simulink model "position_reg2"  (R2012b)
settings: Solver=ode45  StartTime=0.0  StopTime=10.0  RelTol=1e-3
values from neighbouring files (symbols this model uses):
  D = 10    [position_reg_1.m]    (also in position_reg_2.m; rad_aufhaeng_3.m = [0;ct]; rad_aufhaeng_4.m = [0;ct])
  FG = 500    [coulomb_1.m]    (also in coulomb_10.m = 10; coulomb_11.m = 10; coulomb_2.m; coulomb_3.m)
  FH = 12    [coulomb_10.m]    (also in coulomb_11.m; coulomb_3.m = 600; coulomb_4.m = 600; position_reg_1.m = 3.956)
  I = 20    [position_reg_1.m]    (also in position_reg_2.m; suspension_1.m = 225; suspension_2.m = 225; suspension_3.m = 225)
  m1 = 100    [feder_masse_1.m]    (also in feder_masse_11.m; feder_masse_13.m; feder_masse_14.m; position_reg_2.m = 1)
  P = 10    [position_reg_1.m]    (also in position_reg_2.m; vibration_control_1.m = em_ampl*i_ampl/2,; vibration_control_2.m = emf_ampl*i_ampl/2,; vibration_control_3.m = emf_ampl*i_ampl/2,)
  sigma_0 = 5000    [position_reg_1.m]    (also in position_reg_2.m; slip_stick_21.m = 10000; slip_stick_s_12.m = 10000; tilger_gleitreib2.m = 1000)
  sigma_1 = sqrt(sigma_0)    [position_reg_1.m]    (also in position_reg_2.m; slip_stick_21.m = sqrt(1e5); slip_stick_s_12.m = sqrt(1e5); tilger_gleitreib2.m)
  sigma_2 = 0    [position_reg_1.m]    (also in position_reg_2.m; slip_stick_21.m; slip_stick_s_12.m; tilger_gleitreib2.m)
  vs = 0.05    [position_reg_1.m]    (also in position_reg_2.m; slip_stick_21.m; slip_stick_3.m = 0.01; slip_stick_31.m)
libraries: simulink x1

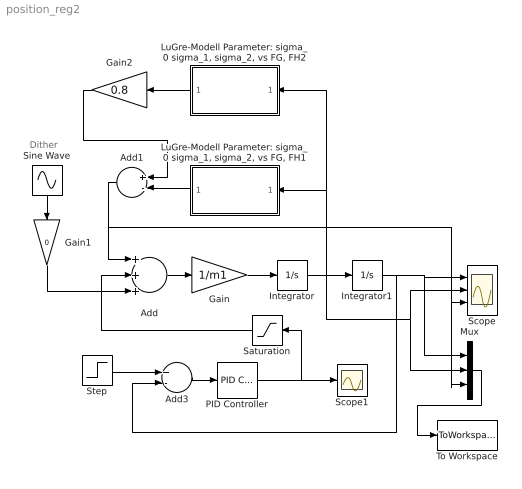
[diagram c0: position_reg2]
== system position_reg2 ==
  note: Dither
  Add : Sum  Inputs=+++
  Add1 : Sum  Inputs=+-
  Add3 : Sum  Inputs=+-
  Gain : Gain  Gain=1/m1
  Gain1 : Gain  Gain=0
  Gain2 : Gain  Gain=0.8
  Integrator : Integrator
  Integrator1 : Integrator
  "LuGre-Modell Parameter: sigma_0 sigma_1, sigma_2, vs FG, FH1" : Subsystem
  "LuGre-Modell Parameter: sigma_0 sigma_1, sigma_2, vs FG, FH2" : Subsystem
  Mux : Mux  Inputs=3
  PID Controller : simulink/Continuous/PID Controller  Controller=PID  TimeDomain=Continuous-time  SampleTime=1  IntegratorMethod=Forward Euler  FilterMethod=Forward Euler  Form=Parallel  P=P  I=I  D=D  N=100  InitialConditionSource=internal  InitialConditionForIntegrator=0  InitialConditionForFilter=0  ExternalReset=none  LimitOutput=off  UpperSaturationLimit=inf  LowerSaturationLimit=-inf  LinearizeAsGain=on  AntiWindupMode=none  Kb=1  TrackingMode=off  Kt=1  PParamMin=[]  PParamMax=[]  IParamMin=[]  IParamMax=[]  DParamMin=[]  DParamMax=[]  NParamMin=[]  NParamMax=[]  KbParamMin=[]  KbParamMax=[]  KtParamMin=[]  KtParamMax=[]  POutMin=[]  POutMax=[]  IOutMin=[]  IOutMax=[]  DOutMin=[]  DOutMax=[]  NOutMin=[]  NOutMax=[]  KbOutMin=[]  KbOutMax=[]  KtOutMin=[]  KtOutMax=[]  IntegratorOutMin=[]  IntegratorOutMax=[]  FilterOutMin=[]  FilterOutMax=[]  SumOutMin=[]  SumOutMax=[]  SumI1OutMin=[]  SumI1OutMax=[]  SumI2OutMin=[]  SumI2OutMax=[]  SumI3OutMin=[]  SumI3OutMax=[]  SumDOutMin=[]  SumDOutMax=[]  SaturationOutMin=[]  SaturationOutMax=[]  IntegratorContinuousStateAttributes=''  IntegratorStateMustResolveToSignalObject=off  IntegratorRTWStateStorageClass=Auto  FilterContinuousStateAttributes=''  FilterStateMustResolveToSignalObject=off  FilterRTWStateStorageClass=Auto
  Saturation : Saturate  UpperLimit=5  LowerLimit=-5  ZeroCross=off
  Scope : Scope  NumInputPorts=3
  Scope1 : Scope
  Sine Wave : Sin  Amplitude=4  Frequency=30  SampleTime=0
  Step : Step  Time=0  SampleTime=0
  To Workspace : ToWorkspace  VariableName=y  SampleTime=-1  SaveFormat=Structure With Time
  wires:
  Add/1 -> Gain/1
  Gain/1 -> Integrator/1
  Integrator/1 -> "LuGre-Modell Parameter: sigma_0 sigma_1, sigma_2, vs FG, FH1"/1(v), "LuGre-Modell Parameter: sigma_0 sigma_1, sigma_2, vs FG, FH2"/1(v), Mux/2, Scope/2, Integrator1/1
  Integrator1/1 -> Add3/2, Mux/1, Scope/1
  Add3/1 -> PID Controller/1
  Step/1 -> Add3/1
  "LuGre-Modell Parameter: sigma_0 sigma_1, sigma_2, vs FG, FH1"/1(Fr) -> Add1/2
  PID Controller/1 -> Saturation/1, Scope1/1
  Saturation/1 -> Add/2
  Sine Wave/1 -> Gain1/1
  Mux/1 -> To Workspace/1
  Gain1/1 -> Add/3
  "LuGre-Modell Parameter: sigma_0 sigma_1, sigma_2, vs FG, FH2"/1(Fr) -> Gain2/1
  Gain2/1 -> Add1/1
  Add1/1 -> Scope/3, Mux/3, Add/1

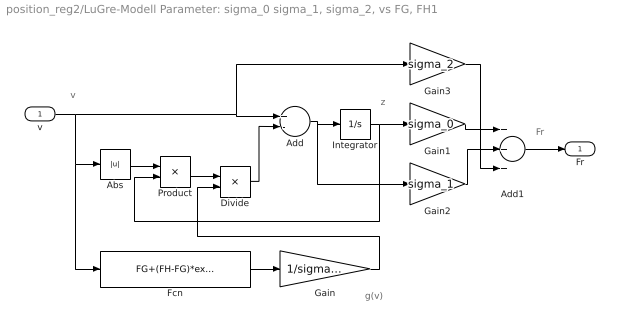
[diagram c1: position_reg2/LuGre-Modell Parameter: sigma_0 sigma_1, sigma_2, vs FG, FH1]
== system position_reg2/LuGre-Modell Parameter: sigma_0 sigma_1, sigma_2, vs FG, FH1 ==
  note: Fr
  note: v
  note: g(v)
  note: z
  v : Inport
  Abs : Abs
  Add : Sum  Inputs=+-
  Add1 : Sum  Inputs=+++
  Divide : Product  Inputs=*/
  Fcn : Fcn  Expr=FG+(FH-FG)*exp(-(u/vs)^2)
  Gain : Gain  Gain=1/sigma_0
  Gain1 : Gain  Gain=sigma_0
  Gain2 : Gain  Gain=sigma_1
  Gain3 : Gain  Gain=sigma_2
  Integrator : Integrator  ZeroCross=off
  Product : Product
  Fr : Outport
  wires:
  v/1 -> Gain3/1, Add/1, Abs/1, Fcn/1
  Integrator/1 -> Gain1/1, Product/2
  Add/1 -> Gain2/1, Integrator/1
  Gain2/1 -> Add1/2
  Abs/1 -> Product/1
  Divide/1 -> Add/2
  Gain1/1 -> Add1/1
  Add1/1 -> Fr/1
  Gain3/1 -> Add1/3
  Fcn/1 -> Gain/1
  Gain/1 -> Divide/2
  Product/1 -> Divide/1

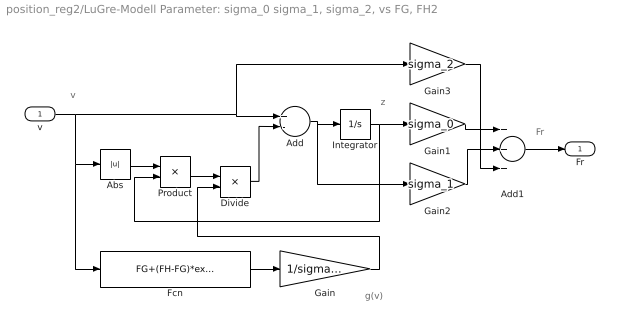
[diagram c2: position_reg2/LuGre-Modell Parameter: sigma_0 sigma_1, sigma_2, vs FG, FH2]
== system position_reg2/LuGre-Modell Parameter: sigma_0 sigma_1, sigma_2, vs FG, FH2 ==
  note: z
  note: g(v)
  note: v
  note: Fr
  v : Inport
  Abs : Abs
  Add : Sum  Inputs=+-
  Add1 : Sum  Inputs=+++
  Divide : Product  Inputs=*/
  Fcn : Fcn  Expr=FG+(FH-FG)*exp(-(u/vs)^2)
  Gain : Gain  Gain=1/sigma_0
  Gain1 : Gain  Gain=sigma_0
  Gain2 : Gain  Gain=sigma_1
  Gain3 : Gain  Gain=sigma_2
  Integrator : Integrator  ZeroCross=off
  Product : Product
  Fr : Outport
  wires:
  Product/1 -> Divide/1
  Gain/1 -> Divide/2
  Fcn/1 -> Gain/1
  Gain3/1 -> Add1/3
  Add1/1 -> Fr/1
  Gain1/1 -> Add1/1
  Divide/1 -> Add/2
  Abs/1 -> Product/1
  Gain2/1 -> Add1/2
  Add/1 -> Integrator/1, Gain2/1
  Integrator/1 -> Product/2, Gain1/1
  v/1 -> Fcn/1, Abs/1, Add/1, Gain3/1
